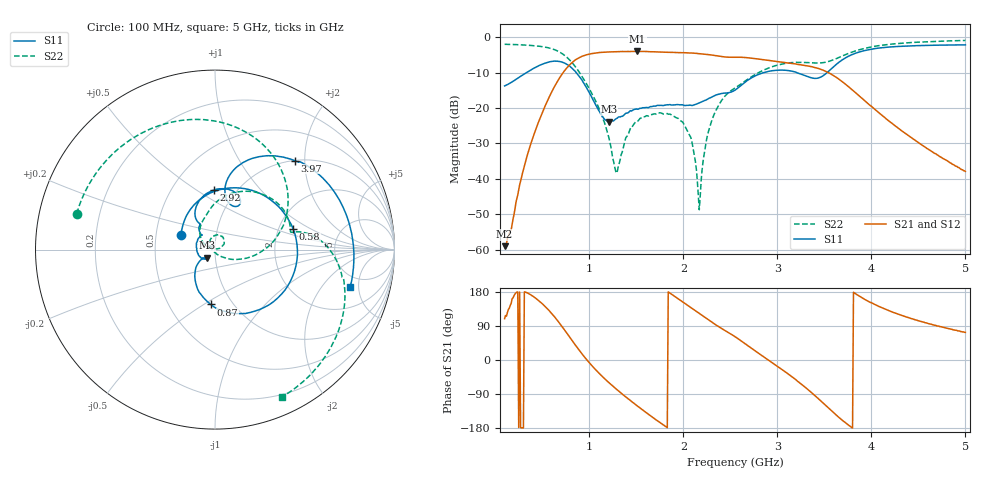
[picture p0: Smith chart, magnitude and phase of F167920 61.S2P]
!  2-Port S-parameters saved by WinCal
! VAR MeasName=S-Parameters (CALIBRATED_DATA) read from VNA (N5242A)
! VAR MeasDate=2016-11-22 9:58:34
! VAR NAME=F167920 61
! VAR FILENAME=F167920 61.S2P
! VAR DATE=2016-11-22 9:58:34
! VAR PHYS_PORTS=1,2
# Hz S DB R 50
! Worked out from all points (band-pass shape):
!   491 points, 100 MHz to 5 GHz, reference 50 ohm
!   highest |S21| = -3.98 dB at 1.51 GHz (marker M1); lowest = -59.0 dB at 100 MHz (marker M2)
!   |S21| within 3 dB of the highest: 825.3 MHz to 3.03 GHz (2.204 GHz wide, 114 % of centre)
!   lowest |S11| = -23.9 dB at 1.21 GHz (marker M3), VSWR 1.14, Z = 45.5 - j4.14 ohm
!   |S11| at or under -10 dB: start of sweep to 330.2 MHz; 862.6 MHz to 2.853 GHz (1.99 GHz wide, 107 % of centre); 3.208 GHz to 3.529 GHz (320.7 MHz wide, 9.52 % of centre)
!   |S22| runs from -48.7 to -0.9 dB; largest |S21 - S12| = 0.0009
!   S11 on the Smith chart (normalised r, x): 100 MHz: 0.67, +0.11; 580 MHz: 2.41, +0.68; 870 MHz: 0.79, -0.54; 2.92 GHz: 0.79, +0.59; 3.97 GHz: 1.01, +1.79; 5 GHz: 3.72, -3.99
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1e8  -13.75 157.2  -59.01 109.3  -59.94 109.4  -1.98 165.5
4e8  -8.90 73.6  -28.41 168.6  -28.40 168.3  -2.34 119.0
5.8e8  -6.92 14.5  -16.56 128.6  -16.56 128.6  -3.08 84.1
7.5e8  -7.46 -49.3  -9.03 74.9  -9.02 75.0  -5.37 42.5
8.7e8  -10.27 -94.4  -6.11 33.4  -6.10 33.4  -8.95 12.5
9.2e8  -11.95 -110.6  -5.41 17.2  -5.39 17.2  -10.96 1.2
1.05e9  -18.17 -140.7  -4.51 -21.0  -4.52 -21.0  -17.02 -22.6
1.21e9  -23.88 -134.9  -4.14 -60.0  -4.14 -60.0  -28.48 -57.3
1.29e9  -22.95 -132.6  -4.07 -77.2  -4.07 -77.3  -38.39 -141.6
1.51e9  -20.31 -165.5  -3.98 -121.0  -3.98 -121.0  -23.64 108.1
1.74e9  -19.26 159.4  -4.14 -162.9  -4.14 -162.9  -21.35 74.8
2.06e9  -19.22 132.1  -4.43 141.8  -4.44 141.7  -27.36 25.2
2.17e9  -18.54 132.3  -4.63 122.5  -4.63 122.5  -48.73 84.9
2.24e9  -17.75 130.9  -4.80 110.6  -4.80 110.5  -30.07 162.7
2.3e9  -16.95 128.7  -5.00 100.3  -5.01 100.3  -23.79 153.1
2.55e9  -14.94 121.7  -5.63 61.6  -5.64 61.5  -14.32 106.2
2.92e9  -9.57 90.9  -6.59 -2.8  -6.61 -2.8  -8.55 60.5
3.37e9  -11.51 64.4  -8.34 -87.4  -8.34 -87.4  -7.22 15.1
3.62e9  -7.83 79.6  -11.19 -143.9  -11.20 -143.9  -6.11 11.3
3.97e9  -3.53 48.0  -18.86 154.5  -18.89 154.4  -2.89 -10.7
4.19e9  -2.76 30.6  -23.73 129.8  -23.72 130.0  -2.00 -25.5
5e9  -2.14 -15.5  -37.90 72.9  -38.00 72.9  -0.90 -65.6
